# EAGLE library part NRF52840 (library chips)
ultra-low power 2.4 GHz wireless system on chip (SoC) integrating a multiprotocol 2.4 GHz transceiver, an ARM® Cortex®-M4F CPU.
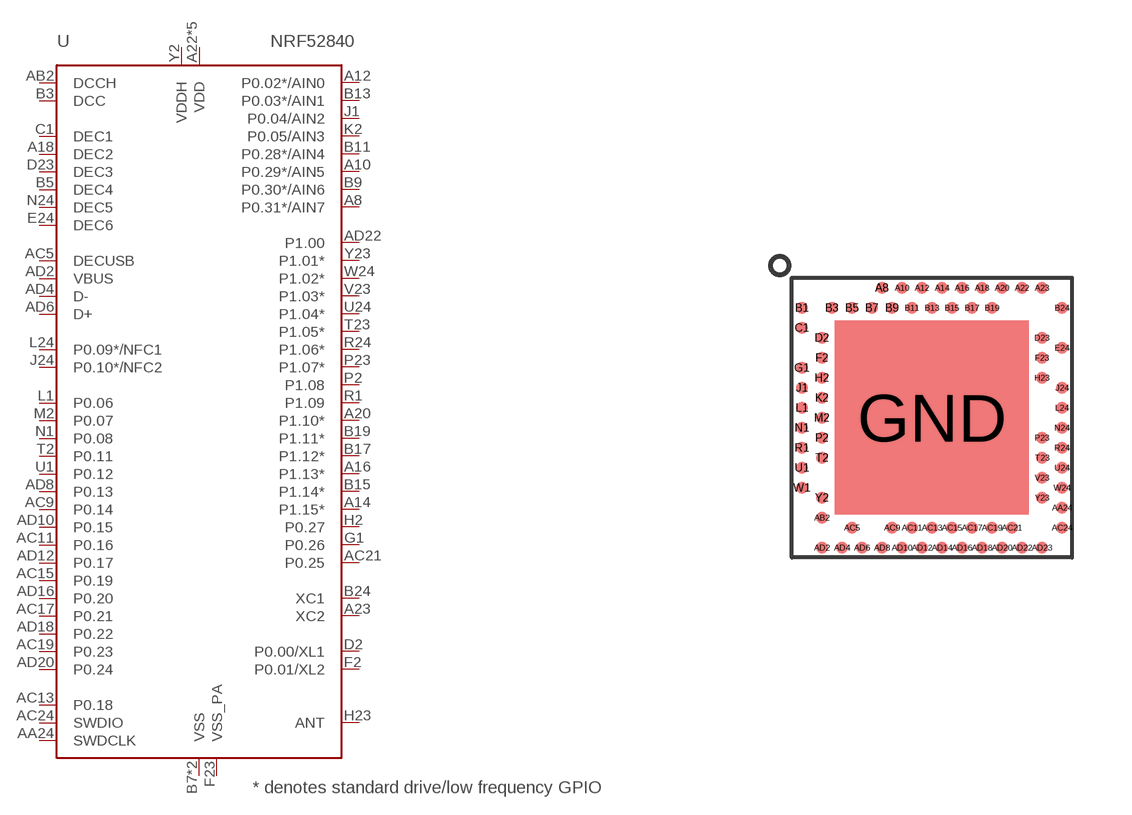
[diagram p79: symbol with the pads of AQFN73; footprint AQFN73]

Designator prefix U

## NRF52840 (DIGIKEY: 1490-1071-1-ND; MANUFACTURER: NORIDIC SEMICONDUCTOR; MPN: NRF52840)  [AQFN73]
A8  P0.31*/AIN7
A10  P0.29*/AIN5
A12  P0.02*/AIN0
A14  P1.15*
A16  P1.13*
A18  DEC2
A20  P1.10*
A22  VDD
A23  XC2
AA24  SWDCLK
AB2  DCCH
AC5  DECUSB
AC9  P0.14
AC11  P0.16
AC13  P0.18
AC15  P0.19
AC17  P0.21
AC19  P0.23
AC21  P0.25
AC24  SWDIO
AD2  VBUS
AD4  D-
AD6  D+
AD8  P0.13
AD10  P0.15
AD12  P0.17
AD14  VDD
AD16  P0.20
AD18  P0.22
AD20  P0.24
AD22  P1.00
AD23  VDD
B1  VDD
B3  DCC
B5  DEC4
B7  VSS
B9  P0.30*/AIN6
B11  P0.28*/AIN4
B13  P0.03*/AIN1
B15  P1.14*
B17  P1.12*
B19  P1.11*
B24  XC1
C1  DEC1
D2  P0.00/XL1
D23  DEC3
E24  DEC6
F2  P0.01/XL2
F23  VSS_PA
G1  P0.26
GND  VSS
H2  P0.27
H23  ANT
J1  P0.04/AIN2
J24  P0.10*/NFC2
K2  P0.05/AIN3
L1  P0.06
L24  P0.09*/NFC1
M2  P0.07
N1  P0.08
N24  DEC5
P2  P1.08
P23  P1.07*
R1  P1.09
R24  P1.06*
T2  P0.11
T23  P1.05*
U1  P0.12
U24  P1.04*
V23  P1.03*
W1  VDD
W24  P1.02*
Y2  VDDH
Y23  P1.01*

## Footprint AQFN73 (pad centres in mm)
AQFN73 7x7mm
smd 0.3 x 0.3: A8 -1.25,3.25; A10 -0.75,3.25; A12 -0.25,3.25; A14 0.25,3.25; A16 0.75,3.25; A18 1.25,3.25; A20 1.75,3.25; A22 2.25,3.25; A23 2.75,3.25; AA24 3.25,-2.25; AB2 -2.75,-2.5; AC5 -2,-2.75; AC9 -1,-2.75; AC11 -0.5,-2.75; AC13 0,-2.75; AC15 0.5,-2.75; AC17 1,-2.75; AC19 1.5,-2.75; AC21 2,-2.75; AC24 3.25,-2.75; AD2 -2.75,-3.25; AD4 -2.25,-3.25; AD6 -1.75,-3.25; AD8 -1.25,-3.25; AD10 -0.75,-3.25; AD12 -0.25,-3.25; AD14 0.25,-3.25; AD16 0.75,-3.25; AD18 1.25,-3.25; AD20 1.75,-3.25; AD22 2.25,-3.25; AD23 2.75,-3.25; B1 -3.25,2.75; B3 -2.5,2.75; B5 -2,2.75; B7 -1.5,2.75; B9 -1,2.75; B11 -0.5,2.75; B13 0,2.75; B15 0.5,2.75; B17 1,2.75; B19 1.5,2.75; B24 3.25,2.75; C1 -3.25,2.25; D2 -2.75,2; D23 2.75,2; E24 3.25,1.75; F2 -2.75,1.5; F23 2.75,1.5; G1 -3.25,1.25; H2 -2.75,1; H23 2.75,1; J1 -3.25,0.75; J24 3.25,0.75; K2 -2.75,0.5; L1 -3.25,0.25; L24 3.25,0.25; M2 -2.75,0; N1 -3.25,-0.25; N24 3.25,-0.25; P2 -2.75,-0.5; P23 2.75,-0.5; R1 -3.25,-0.75; R24 3.25,-0.75; T2 -2.75,-1; T23 2.75,-1; U1 -3.25,-1.25; U24 3.25,-1.25; V23 2.75,-1.5; W1 -3.25,-1.75; W24 3.25,-1.75; Y2 -2.75,-2; Y23 2.75,-2
smd 4.85 x 4.85: GND 0,0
